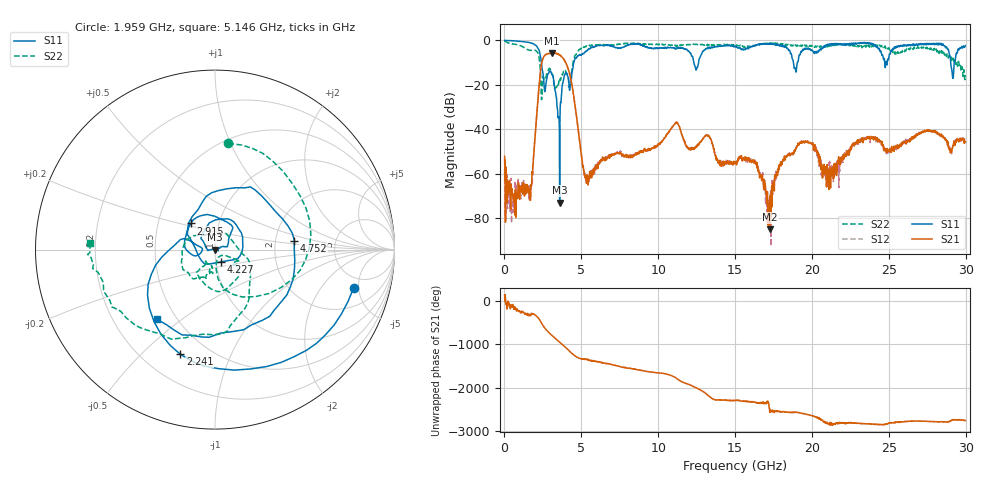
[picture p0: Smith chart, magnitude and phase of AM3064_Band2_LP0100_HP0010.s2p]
# Hz S DB R 50.0
!freq dBS11 angS11 dBS21 angS21 dBS12 angS12 dBS22 angS22
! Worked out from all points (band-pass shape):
!   1600 points, 10 MHz to 29.98 GHz, reference 50 ohm
!   highest |S21| = -5.69 dB at 3.084 GHz (marker M1); lowest = -85.1 dB at 17.29 GHz (marker M2)
!   |S21| within 3 dB of the highest: 2.479 GHz to 3.881 GHz (1.402 GHz wide, 44.1 % of centre)
!   lowest |S11| = -73.0 dB at 3.59 GHz (marker M3), VSWR 1.00, Z = 50 + j0.0171 ohm
!   |S11| at or under -10 dB: 2.402 GHz to 4.507 GHz (2.105 GHz wide, 60.9 % of centre); 12.31 GHz to 12.62 GHz (308.4 MHz wide, 2.47 % of centre); 18.8 GHz to 19.05 GHz (252.5 MHz wide, 1.33 % of centre)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
!   |S22| runs from -26.7 to -0.2 dB; largest |S21 - S12| = 0.016
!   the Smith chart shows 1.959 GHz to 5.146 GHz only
!   S11 on the Smith chart (normalised r, x): 1.959 GHz: 3.69, -4.38; 2.241 GHz: 0.35, -0.66; 2.915 GHz: 0.73, +0.22; 4.227 GHz: 1.06, -0.15; 4.752 GHz: 2.56, +0.32; 5.146 GHz: 0.39, -0.41
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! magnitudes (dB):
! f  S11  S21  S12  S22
! 10 MHz  0.0  -52.2  -58.3  -0.2
! 1.566 GHz  -0.9  -66.6  -65.0  -4.3
! 1.959 GHz  -1.9  -46.3  -46.1  -4.5
! 2.241 GHz  -4.2  -21.5  -21.5  -7.5
! 2.915 GHz  -14.0  -6.0  -5.9  -12.7
! 3.084 GHz  -15.4  -5.7  -5.7  -14.9
! 3.59 GHz  -73.0  -6.6  -6.6  -17.0
! 4.227 GHz  -22.4  -14.8  -14.7  -20.9
! 4.752 GHz  -7.0  -37.8  -37.9  -5.1
! 5.015 GHz  -6.6  -52.4  -52.4  -3.8
! 5.146 GHz  -5.9  -58.4  -57.9  -3.2
! 10 GHz  -3.5  -47.1  -47.1  -1.8
! 11.18 GHz  -3.4  -37.1  -36.9  -2.5
! 15 GHz  -2.6  -54.9  -55.3  -2.0
! 16.26 GHz  -2.4  -54.5  -54.4  -2.5
! 17.29 GHz  -1.7  -85.1  -69.8  -1.3
! 18.1 GHz  -2.5  -54.6  -54.1  -1.4
! 19.99 GHz  -4.4  -46.6  -46.3  -2.3
! 21.08 GHz  -2.4  -58.4  -57.7  -2.3
! 23.14 GHz  -1.1  -45.4  -44.5  -3.2
! 25 GHz  -8.0  -49.9  -49.5  -3.3
! 29.98 GHz  -2.4  -45.7  -45.8  -15.8
